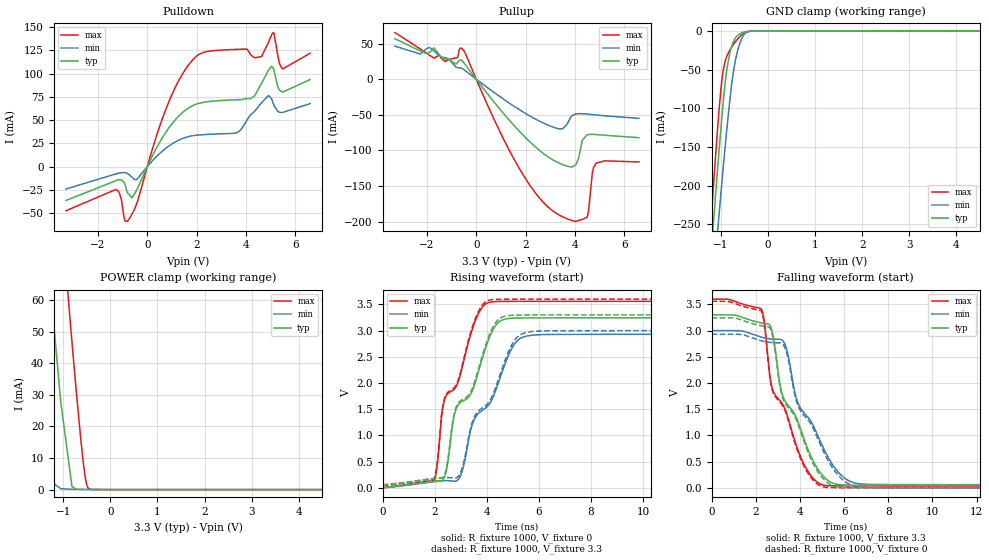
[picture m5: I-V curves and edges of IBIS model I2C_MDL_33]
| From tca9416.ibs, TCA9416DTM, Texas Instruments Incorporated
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[Model]   I2C_MDL_33
Model_type   I/O
Polarity   Non-Inverting
Enable   Active-High
Vinl = 0.99
Vinh = 2.41
Vmeas = 1.65
Vref = 0
Cref = 2pF
Rref = 100000
|   typ   min   max
C_comp   7.2608pF   6.6746pF   7.8469pF
[Voltage Range]   3.3   3   3.6
[Temperature Range]   27   125   -40
[Pullup Reference]   3.3   3   3.6
[Pulldown Reference]   0   -0   0
[Power Clamp Reference]   3.3   3   3.6
[GND Clamp Reference]   0   0   0
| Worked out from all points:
|   slope of the pulldown table from 0 to 0.495 V, typ, clamps not added: 19.1 ohm
|   slope of the pullup table from 0 to 0.495 V, typ, clamps not added: 22.3 ohm
|   GND clamp passes 1 mA (typ) near -0.46 V on its own axis
|   POWER clamp passes 1 mA (typ) near -0.82 V on its own axis
|   rising waveform, R_fixture 1000, V_fixture 0: 20-80 % time 1.36ns typ, 1.5ns min, 1.18ns max; typ from 0.001 V to 3.24 V
|   falling waveform, R_fixture 1000, V_fixture 3.3: 20-80 % time 1.52ns typ, 1.68ns min, 1.43ns max; typ from 3.3 V to 0.049 V
|   rising waveform, R_fixture 1000, V_fixture 3.3: 20-80 % time 1.36ns typ, 1.5ns min, 1.18ns max; typ from 0.049 V to 3.3 V
|   falling waveform, R_fixture 1000, V_fixture 0: 20-80 % time 1.52ns typ, 1.67ns min, 1.43ns max; typ from 3.24 V to 0.001 V
[Pulldown]
|I2C_MDL_33
|   Voltage   I(typ)   I(min)   I(max)
-3.3V     -36.37mA   -24.11mA   -47.41mA
-1.28V    -15.2mA    -7.899mA   -24.63mA
-805.2mV  -28.19mA   -7.403mA   -58.81mA
-518.1mV  -29.33mA   -14.02mA   -45.67mA
986.7mV   45.6mA     24.17mA    76.85mA
2.095V    68.02mA    33.94mA    120.6mA
3.64V     71.84mA    36.5mA     126mA
4.165V    72.71mA    54.94mA    120.7mA
4.63V     89.26mA    68.49mA    118.2mA
5.036V    107.6mA    73.19mA    141.3mA
5.501V    80.15mA    58.24mA    105.1mA
6.6V      93.53mA    67.71mA    121.7mA
[GND Clamp]
|I2C_MDL_33
|   Voltage   I(typ)   I(min)   I(max)
-3.3V     -2.028A    -1.856A    -2.21A
-1.389V   -435.6mA   -488.2mA   -409.1mA
-1.171V   -257.3mA   -330.5mA   -210.8mA
-1.162V   -249.3mA   -323.4mA   -202.1mA
-1.082V   -186.7mA   -266.9mA   -134.8mA
-1.043V   -156.3mA   -239mA     -103.9mA
-973.5mV  -106.3mA   -191.1mA   -60.33mA
-874.5mV  -49.39mA   -126.3mA   -32.31mA
-726mV    -12.65mA   -49.26mA   -16.69mA
-537.9mV  -2.24mA    -7.555mA   -4.282mA
-250.8mV  -348.1uA   -301.6uA   -423.1uA
6.6V      0A         0A         0A
[Pullup]
|I2C_MDL_33
|   Voltage   I(typ)   I(min)   I(max)
-3.3V     56.92mA    46.31mA    65.42mA
-1.894V   37.56mA    44.51mA    33.59mA
-1.261V   28.24mA    30.05mA    24.65mA
-528mV    24.1mA     13.92mA    40.98mA
1.818V    -75.65mA   -44.25mA   -129.4mA
3.482V    -119.6mA   -69.78mA   -192.8mA
4.036V    -120.3mA   -48.88mA   -199.5mA
4.303V    -85.75mA   -48.52mA   -196.9mA
4.491V    -78.33mA   -49.02mA   -194mA
4.709V    -77.49mA   -49.77mA   -131.8mA
4.867V    -77.75mA   -50.32mA   -117.8mA
6.6V      -82.18mA   -55.03mA   -116.2mA
[POWER Clamp]
|I2C_MDL_33
|   Voltage   I(typ)   I(min)   I(max)
-3.3V     1.443A     1.132A     1.766A
-1.676V   137.7mA    67.99mA    246.7mA
-1.607V   124.6mA    56.24mA    209.2mA
-1.35V    78.35mA    16.27mA    143.5mA
-1.181V   49.07mA    1.635mA    112.4mA
-1.053V   27.79mA    280.5uA    88.94mA
-815.1mV  986.4uA    100.5uA    46.85mA
-666.6mV  85.37uA    64.55uA    22.06mA
-567.6mV  54.86uA    49.62uA    7.733mA
-508.2mV  47.11uA    42.96uA    1.965mA
-448.8mV  40.87uA    37.16uA    208.6uA
6.6V      0A         0A         0A
[Ramp]
| I2C_MDL_33
| variable   typ   min   max
dV/dt_r   1.95/1.36E-09   1.76/1.50E-09   2.13/1.19E-09
dV/dt_f   1.95/1.52E-09   1.76/1.68E-09   2.14/1.43E-09
R_load = 1000
[Rising Waveform]
| IOADSB_33
R_fixture =   1000
C_fixture =   0
L_fixture =   0
V_fixture =   0
V_fixture_min = 0
V_fixture_max = 0
|   Time   V(typ)   V(min)   V(max)
0s        1.202mV    1.292mV    1.029mV
1.985ns   131.3mV    117.6mV    150mV
2.337ns   170.3mV    136.3mV    1.611V
2.821ns   1.506V     132mV      1.935V
3.349ns   1.767V     1.035V     2.876V
3.657ns   2.184V     1.412V     3.304V
4.361ns   3.113V     1.891V     3.554V
5.153ns   3.24V      2.8V       3.557V
6.429ns   3.243V     2.926V     3.558V
219.8ns   3.244V     2.93V      3.559V
[Falling Waveform]
|I2C_MDL_33
R_fixture =   1000
C_fixture =   0
L_fixture =   0
V_fixture =   3.3
V_fixture_min = 3
V_fixture_max = 3.6
|   Time   V(typ)   V(min)   V(max)
0s        3.3V       3V         3.6V
2.249ns   3.147V     2.877V     3.416V
2.645ns   3.099V     2.842V     2.126V
3.261ns   1.71V      2.789V     1.562V
3.921ns   1.253V     1.612V     711.7mV
4.625ns   493.3mV    1.171V     170.8mV
5.373ns   114.5mV    514.6mV    41.24mV
6.341ns   53.12mV    112mV      37.06mV
8.057ns   50.13mV    63.42mV    36.22mV
219.8ns   49.46mV    61.38mV    35.9mV
[Rising Waveform]
|I2C_MDL_33
R_fixture =   1000
C_fixture =   0
L_fixture =   0
V_fixture =   3.3
V_fixture_min = 3
V_fixture_max = 3.6
|   Time   V(typ)   V(min)   V(max)
0s        49.46mV    61.38mV    35.9mV
1.985ns   180.3mV    178.5mV    185.4mV
2.337ns   219.1mV    196.9mV    1.639V
2.821ns   1.542V     191.4mV    1.968V
3.349ns   1.806V     1.091V     2.917V
3.657ns   2.236V     1.457V     3.345V
4.361ns   3.168V     1.953V     3.596V
5.153ns   3.296V     2.869V     3.599V
6.429ns   3.299V     2.997V     3.599V
219.8ns   3.3V       3V         3.6V
[Falling Waveform]
|I2C_MDL_33
R_fixture =   1000
C_fixture =   0
L_fixture =   0
V_fixture =   0
V_fixture_min = 0
V_fixture_max = 0
|   Time   V(typ)   V(min)   V(max)
0s        3.244V     2.93V      3.559V
2.249ns   3.093V     2.808V     3.377V
2.645ns   3.045V     2.775V     2.09V
3.261ns   1.671V     2.722V     1.532V
3.833ns   1.303V     1.665V     779.9mV
4.273ns   785.3mV    1.341V     344.8mV
5.373ns   66.12mV    451.6mV    6.346mV
6.341ns   4.861mV    51.46mV    2.183mV
8.057ns   1.872mV    3.323mV    1.351mV
219.8ns   1.202mV    1.292mV    1.029mV
